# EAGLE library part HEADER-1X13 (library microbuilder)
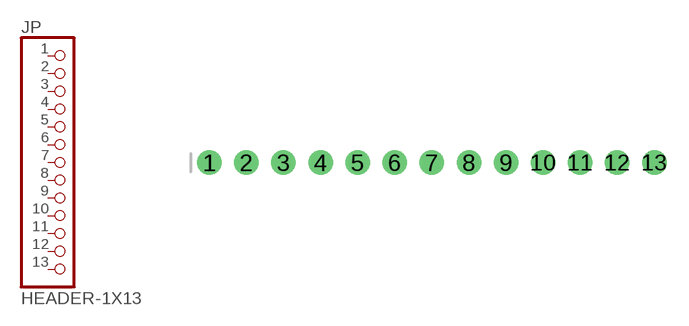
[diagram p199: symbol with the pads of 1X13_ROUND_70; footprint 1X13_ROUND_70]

Designator prefix JP

## HEADER-1X13  [1X13_ROUND_70]
1  1  pas
2  2  pas
3  3  pas
4  4  pas
5  5  pas
6  6  pas
7  7  pas
8  8  pas
9  9  pas
10  10  pas
11  11  pas
12  12  pas
13  13  pas

## Footprint 1X13_ROUND_70 (pad centres in mm)
drill 1 pad 1.676: 1 -15.24,0; 2 -12.7,0; 3 -10.16,0; 4 -7.62,0; 5 -5.08,0; 6 -2.54,0; 7 0,0; 8 2.54,0; 9 5.08,0; 10 7.62,0; 11 10.16,0; 12 12.7,0; 13 15.24,0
